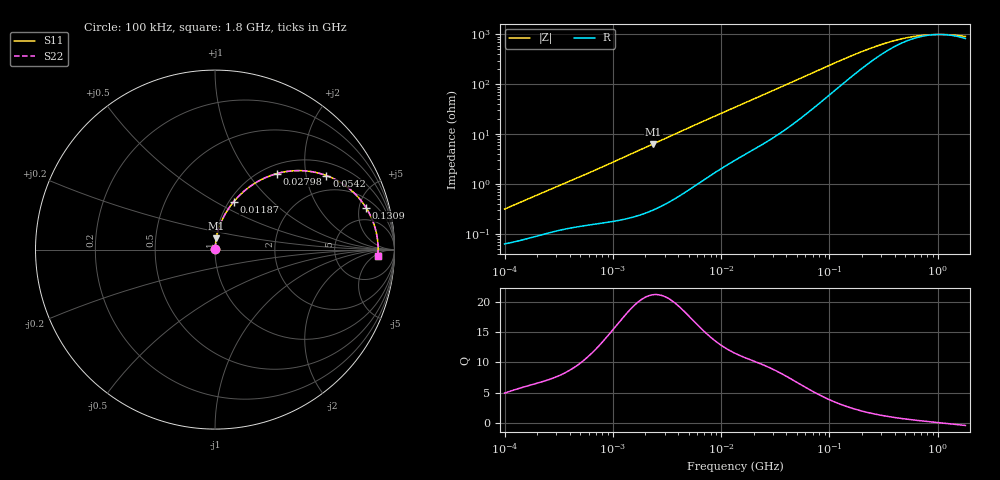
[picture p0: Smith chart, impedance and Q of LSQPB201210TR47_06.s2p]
! LSQPB201210TR47_06  S-PARAMETER MODEL  ( General Type )
! Model Generated by TAIYO YUDEN Corporation (http://www.ty-top.com)
! Version 1.0
! TAIYO YUDEN Control No. 120417NG38SB-FKC
! Copyright(c) 2012 TAIYO YUDEN CO.,LTD. All Rights Reserved.
! Product Description (link to TY-COMPAS)
! https://ds.yuden.co.jp/TYCOMPAS/or/detail?pn=LSQPB201210TR47M06&u=M
! Products Name : Inductors
! Characteristics :
!  Inductance : 0.47 uH , SRF(min) : 500 MHz , DC Resistance(max) : 0.0624 Ohm
!  Rated Current : Saturation :1500 mA , Temp Rise : 1900 mA (40 degC)
!  Case Size : 2.0 x 1.25 / 0.079 x 0.049 [mm/inch] , Thickness : 1.0 / 0.04 [mm/inch]
!  (Conditions: Temperature = 25 degC , DC Bias Current/Voltage = 0A / 0V)
! External Node Assignments :
!  1  o---GGG---o  2
! GND o---------o GND
! Frequency Range : 0.1MHz  -  1800MHz  [ 402 STEP ]
# MHz S RI R 50
! Freq[MHz].  S11 Real  S11 Imag  S21 Real  S21 Imag  S12 Real  S12 Imag  S22 Real  S22 Imag
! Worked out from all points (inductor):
!   401 points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, 100 kHz to 1.8 GHz, reference 50 ohm
!   read as one part in series: L = 486 nH near 105 kHz
!   highest Q = 21.2 at 2.357 MHz (marker M1), where L = 431 nH
!   self-resonance near 1.037 GHz
!   S11 on the Smith chart (normalised r, x): 100 kHz: 1.00, +0.01; 11.87 MHz: 1.05, +0.61; 27.98 MHz: 1.15, +1.39; 54.2 MHz: 1.42, +2.63; 130.9 MHz: 2.99, +5.89; 1.8 GHz: 18, -8
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0.1  0.000638 0.00308  0.9994 -0.00308  0.9994 -0.00308  0.000638 0.00308
0.516129  0.00164 0.0144  0.9984 -0.0144  0.9984 -0.0144  0.00164 0.0144
1.216451  0.00301 0.033  0.997 -0.033  0.997 -0.033  0.00301 0.033
2.356814  0.00702 0.0632  0.993 -0.0632  0.993 -0.0632  0.00702 0.0632
2.66389  0.0085 0.0712  0.9915 -0.0712  0.9915 -0.0712  0.0085 0.0712
4.242694  0.0186 0.1112  0.9814 -0.1112  0.9814 -0.1112  0.0186 0.1112
6.434145  0.0383 0.1627  0.9617 -0.1627  0.9617 -0.1627  0.0383 0.1627
11.86985  0.1052 0.2679  0.8948 -0.2679  0.8948 -0.2679  0.1052 0.2679
13.41641  0.127 0.2923  0.873 -0.2923  0.873 -0.2923  0.127 0.2923
19.37354  0.216 0.3658  0.784 -0.3658  0.784 -0.3658  0.216 0.3658
27.97575  0.3442 0.4234  0.6558 -0.4234  0.6558 -0.4234  0.3442 0.4234
38.46609  0.4783 0.44  0.5217 -0.44  0.5217 -0.44  0.4783 0.44
54.20166  0.6211 0.4125  0.3789 -0.4125  0.3789 -0.4125  0.6211 0.4125
69.24595  0.7068 0.3697  0.2932 -0.3697  0.2932 -0.3697  0.7068 0.3697
95.21179  0.7895 0.301  0.2105 -0.301  0.2105 -0.301  0.7895 0.301
130.9143  0.8423 0.2326  0.1577 -0.2326  0.1577 -0.2326  0.8423 0.2326
213.6735  0.8841 0.1459  0.1159 -0.1459  0.1159 -0.1459  0.8841 0.1459
357.3983  0.9013 0.0819  0.0987 -0.0819  0.0987 -0.0819  0.9013 0.0819
542.0029  0.9067 0.0448  0.0933 -0.0448  0.0933 -0.0448  0.9067 0.0448
802.0705  0.9087 0.0168  0.0913 -0.0168  0.0913 -0.0168  0.9087 0.0168
1186.925  0.909 -0.00873  0.091 0.00873  0.091 0.00873  0.909 -0.00873
1800  0.9075 -0.0374  0.0925 0.0374  0.0925 0.0374  0.9075 -0.0374
